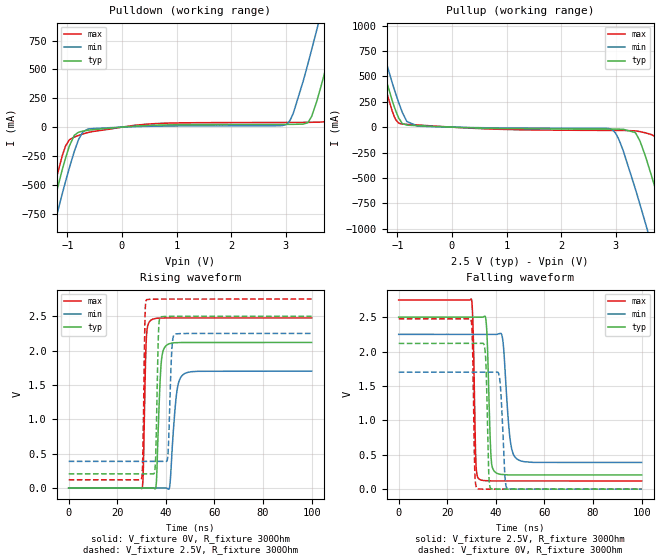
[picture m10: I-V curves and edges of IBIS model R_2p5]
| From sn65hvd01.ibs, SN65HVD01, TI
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|   Model
[Model]   R_2p5
Model_type   Output
Polarity   Non-Inverting
Vmeas = 1.25
Vref = 0
Cref = 1pF
Rref = 100000
|   typ   min   max
C_comp   1pF   1pF   1pF
[Voltage Range]   2.5   2.25   2.75
[Temperature Range]   27   125   -40
[Pullup Reference]   2.5   2.25   2.75
[Pulldown Reference]   -0   -0   -0
[Power Clamp Reference]   2.5   2.25   2.75
[GND Clamp Reference]   -0   -0   -0
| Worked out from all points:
|   slope of the pulldown table from 0 to 0.375 V, typ, clamps not added: 30.6 ohm
|   slope of the pullup table from 0 to 0.375 V, typ, clamps not added: 54.1 ohm
|   falling waveform, V_fixture 2.5V, R_fixture 300Ohm: 20-80 % time 1.18ns typ, 2.22ns min, 866ps max; typ from 2.5 V to 0.207 V
|   rising waveform, V_fixture 0V, R_fixture 300Ohm: 20-80 % time 1.37ns typ, 2.14ns min, 885ps max; typ from 0 V to 2.12 V
|   rising waveform, V_fixture 2.5V, R_fixture 300Ohm: 20-80 % time 813ps typ, 1.04ns min, 666ps max; typ from 0.207 V to 2.5 V
|   falling waveform, V_fixture 0V, R_fixture 300Ohm: 20-80 % time 880ps typ, 1.37ns min, 705ps max; typ from 2.12 V to 0 V
[Pulldown]
|   Voltage   I(typ)   I(min)   I(max)
-2.5V     -3.059A    -3.264A    -2.933A
-1.51V    -1.133A    -1.346A    -1.001A
-1.03V    -261.1mA   -463.4mA   -159.6mA
-790mV    -43.19mA   -101.5mA   -70.83mA
-527.5mV  -21.88mA   -11.88mA   -37.52mA
3.013V    24.07mA    23.48mA    40.9mA
3.41V     39.62mA    549.4mA    41.67mA
3.575V    229.2mA    849mA      42.92mA
3.71V     459.8mA    1.101A     46.83mA
4.01V     1.017A     1.672A     440mA
4.145V    1.275A     1.932A     690.2mA
4.992V    2.926A     3.584A     2.334A
[Pullup]
|   Voltage   I(typ)   I(min)   I(max)
-2.5V     2.941A     3.109A     2.841A
-1.502V   1.003A     1.181A     893.7mA
-977.5mV  90.16mA    242.5mA    38.93mA
-827.5mV  19.57mA    55.93mA    27.33mA
-625mV    14.03mA    9.24mA     20.75mA
2.938V    -19.41mA   -25.63mA   -32.39mA
3.373V    -61.48mA   -625.7mA   -37.48mA
3.553V    -295mA     -955.4mA   -56.95mA
3.665V    -489.7mA   -1.166A    -75.34mA
4.01V     -1.132A    -1.825A    -529.9mA
4.13V     -1.362A    -2.056A    -753mA
4.992V    -3.044A    -3.739A    -2.426A
[Ramp]
R_load = 300
|   typ   min   max
dV/dt_r   1.27103/1.37277e-09   1.02038/2.14082e-09   1.48554/8.84914e-10
dV/dt_f   1.37606/1.17718e-09   1.11729/2.21941e-09   1.57817/8.65825e-10
[Falling Waveform]
V_fixture = 2.5V
V_fixture_min = 2.25V
V_fixture_max = 2.75V
R_fixture = 300Ohm
C_fixture = 0F
|   Time   V(typ)   V(min)   V(max)
0s        2.5V       2.25V      2.75V
29.98ns   2.5V       2.25V      2.759V
31.75ns   2.5V       2.25V      419.6mV
33.21ns   2.5V       2.25V      144.1mV
35.96ns   2.45V      2.25V      123.6mV
38.01ns   471.5mV    2.25V      120.6mV
39.49ns   255.7mV    2.25V      120mV
42.69ns   213.3mV    2.207V     120mV
48.46ns   207.3mV    445.2mV    119.9mV
100ns     206.6mV    387.9mV    119.7mV
[Rising Waveform]
V_fixture = 0V
V_fixture_min = 0V
V_fixture_max = 0V
R_fixture = 300Ohm
C_fixture = 0F
|   Time   V(typ)   V(min)   V(max)
0s        1.049nV    35.32nV    504.6pV
30.2ns    135.7uV    193.7uV    -6.148mV
30.76ns   138.2uV    197.4uV    313.3mV
32.02ns   143.9uV    205.5uV    2.209V
33.93ns   152.5uV    217.7uV    2.445V
35.96ns   26.8mV     230.7uV    2.468V
38.01ns   1.783V     243.8uV    2.473V
39.9ns    2.064V     255.9uV    2.476V
47.17ns   2.118V     1.652V     2.476V
100ns     2.118V     1.701V     2.476V
[Rising Waveform]
V_fixture = 2.5V
V_fixture_min = 2.25V
V_fixture_max = 2.75V
R_fixture = 300Ohm
C_fixture = 0F
|   Time   V(typ)   V(min)   V(max)
0s        206.6mV    387.9mV    119.7mV
29.89ns   206.2mV    387.9mV    125.5mV
32.02ns   206.2mV    387.9mV    2.74V
35.55ns   283.9mV    387.9mV    2.749V
36.92ns   2.206V     387.9mV    2.749V
37.67ns   2.485V     387.9mV    2.75V
40.77ns   2.498V     451.1mV    2.75V
42.45ns   2.499V     2.009V     2.75V
43.57ns   2.499V     2.238V     2.75V
100ns     2.5V       2.25V      2.75V
[Falling Waveform]
|Gnd
V_fixture = 0V
V_fixture_min = 0V
V_fixture_max = 0V
R_fixture = 300Ohm
C_fixture = 0F
|   Time   V(typ)   V(min)   V(max)
0s        2.118V     1.701V     2.476V
29.68ns   2.119V     1.701V     2.47V
30.42ns   2.119V     1.701V     2.068V
31.38ns   2.119V     1.701V     203.7mV
32.3ns    2.119V     1.701V     6.885mV
35.64ns   1.987V     1.701V     442uV
38.01ns   7.214mV    1.701V     204.4uV
41.55ns   690uV      1.608V     192.7uV
44.68ns   310.4uV    9.32mV     182.4uV
100ns     -155.2nV   1.677uV    -13.8nV
